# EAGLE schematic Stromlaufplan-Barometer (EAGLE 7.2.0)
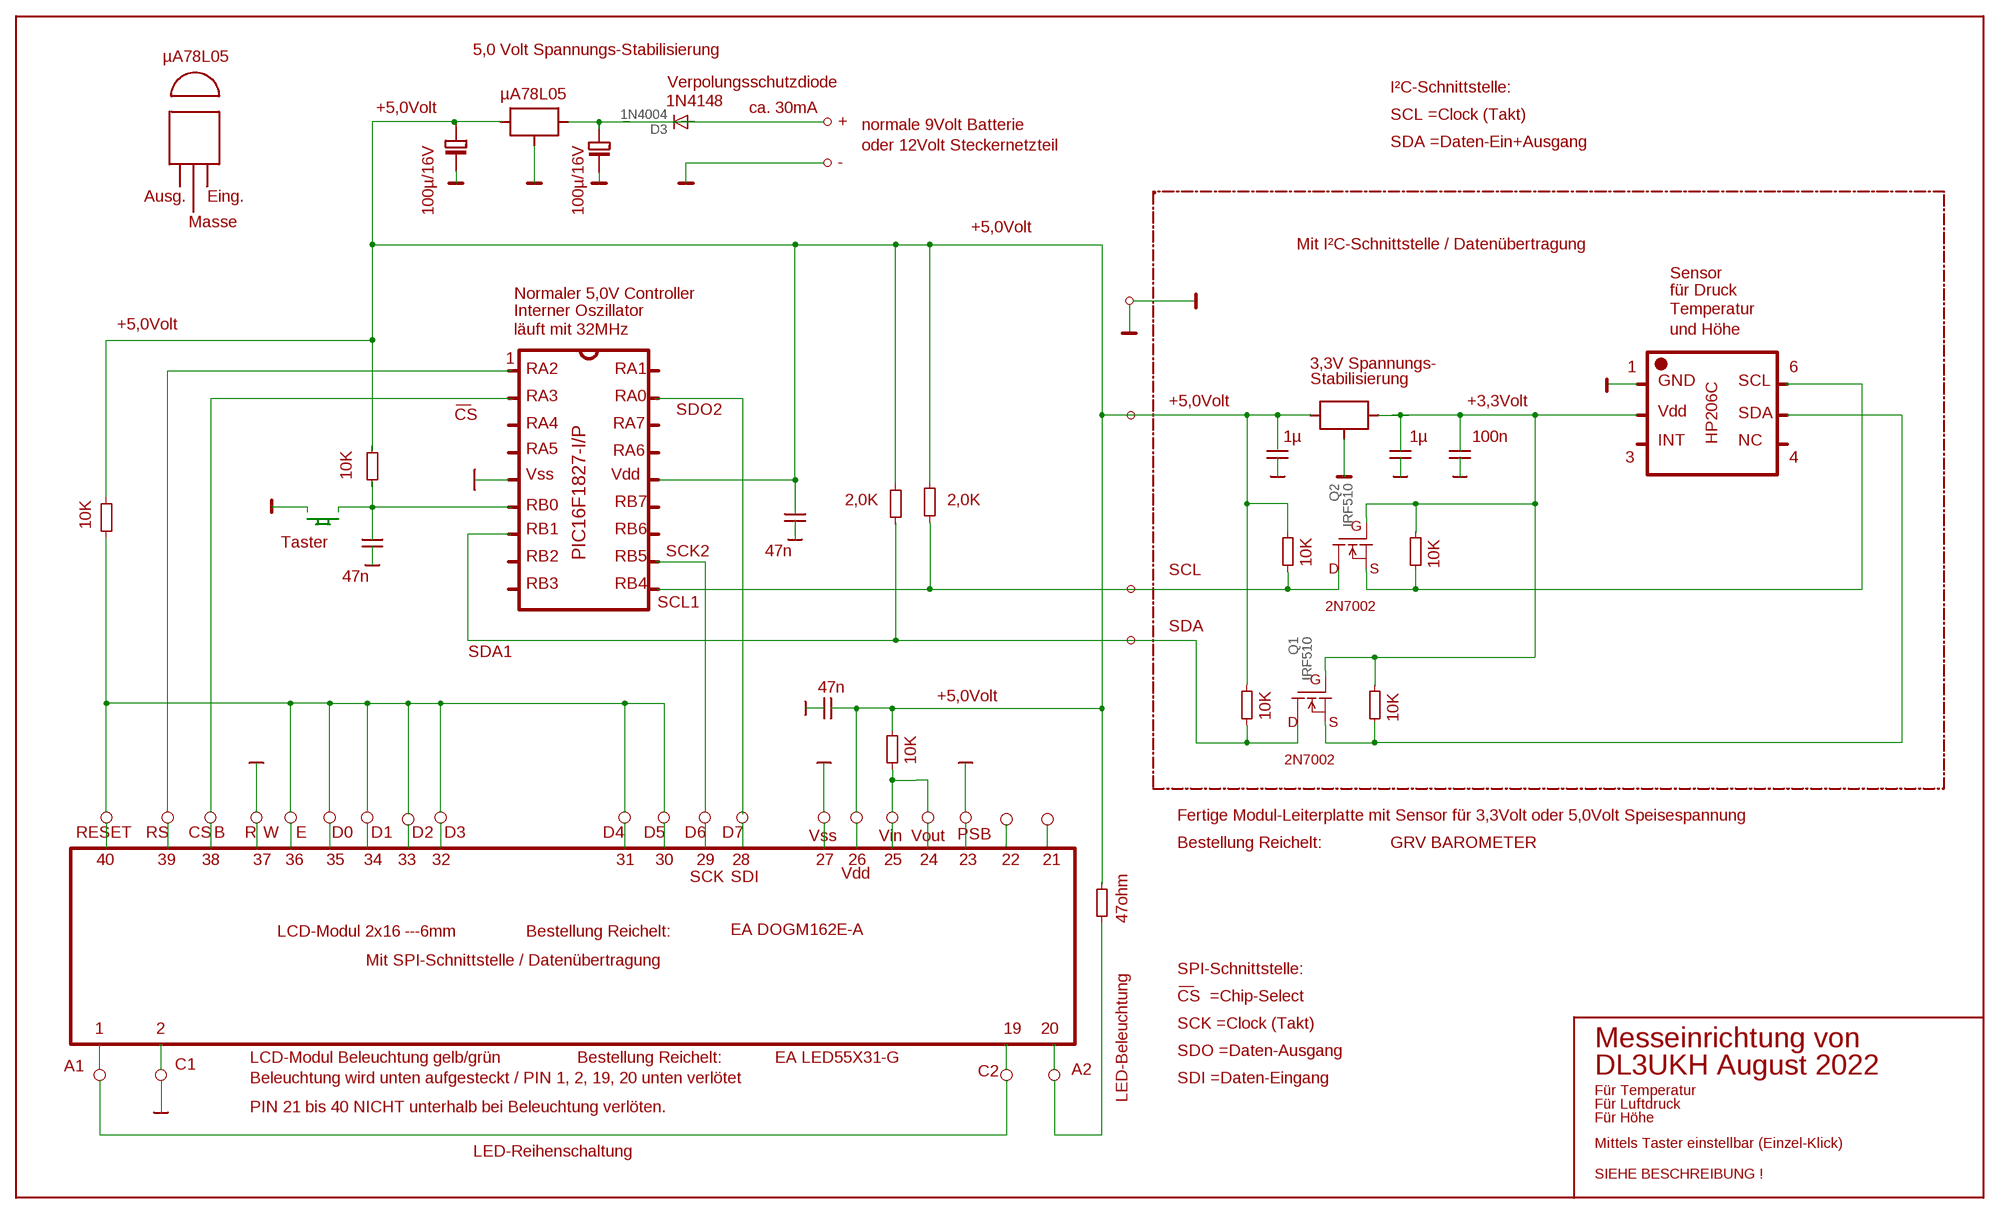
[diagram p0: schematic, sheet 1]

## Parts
D3  1N4004  [DO41-10]
Q1  IRF510  [TO220]
Q2  IRF510  [TO220]

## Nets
N$21: Q2.2(D)
N$22: Q1.3(S)
N$23: Q1.2(D)
N$30: Q1.1(G)
N$35: D3.C
N$47: D3.A
N$55: Q2.1(G)
N$71: Q2.3(S)

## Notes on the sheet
- 5,0 Volt Spannungs-Stabilisierung
- µA78L05
- Verpolungsschutzdiode
- I²C-Schnittstelle:
- µA78L05
- 1N4148
- +5,0Volt | ca. 30mA
- SCL =Clock (Takt)
- + | normale 9Volt Batterie
- oder 12Volt Steckernetzteil | SDA =Daten-Ein+Ausgang
- -
- Ausg. | Eing.
- 100µ/16V | 100µ/16V
- Masse
- +5,0Volt
- Mit I²C-Schnittstelle / Datenübertragung
- Sensor
- Normaler 5,0V Controller | für Druck
- Interner Oszillator | Temperatur
- +5,0Volt
- läuft mit 32MHz | und Höhe
- 1
- 3,3V Spannungs- | 1 | 6
- RA2 | RA1
- Stabilisierung | GND | SCL
- RA3 | RA0
- +5,0Volt | +3,3Volt
- SDO2 | Vdd | SDA
- CS
- RA4 | RA7 | 1µ | 1µ | 100n
- INT | HP206C | NC
- RA5 | RA6
- 3 | 4
- 10K | Vss | Vdd
- RB7 | 2,0K | 2,0K
- RB0
- G
- 10K
- Taster | RB1 | RB6
- 47n
- PIC16F1827-I/P | SCK2
- RB2 | RB5 | D | S
- 47n | 10K | 10K
- SCL
- RB3 | RB4
- 2N7002
- SCL1
- SDA
- SDA1
- G
- 47n
- +5,0Volt
- 10K | D | S
- 10K
- 2N7002
- 10K
- Fertige Modul-Leiterplatte mit Sensor für 3,3Volt oder 5,0Volt Speisespannung
- RESET | RS | CS | B | R | W | E | D0 | D1 | D2 | D3 | D4 | D5 | D6 | D7 | Vss | Vin | Vout | PSB
- Bestellung Reichelt: | GRV BAROMETER
- 40 | 39 | 38 | 37 | 36 | 35 | 34 | 33 | 32 | 31 | 30 | 29 | 28 | 27 | 26 | 25 | 24 | 23 | 22 | 21
- SCK | SDI | Vdd
- 47ohm
- LCD-Modul 2x16 ---6mm | Bestellung Reichelt: | EA DOGM162E-A
- Mit SPI-Schnittstelle / Datenübertragung
- SPI-Schnittstelle:
- CS  =Chip-Select
- SCK =Clock (Takt)
- 1 | 2 | 19 | 20
- Messeinrichtung von
- SDO =Daten-Ausgang
- LCD-Modul Beleuchtung gelb/grün | Bestellung Reichelt: | EA LED55X31-G
- A1 | C1
- C2 | A2 | DL3UKH August 2022
- Beleuchtung wird unten aufgesteckt / PIN 1, 2, 19, 20 unten verlötet | SDI =Daten-Eingang
- Für Temperatur
- LED-Beleuchtung
- PIN 21 bis 40 NICHT unterhalb bei Beleuchtung verlöten. | Für Luftdruck
- Für Höhe
- Mittels Taster einstellbar (Einzel-Klick)
- LED-Reihenschaltung
- SIEHE BESCHREIBUNG !

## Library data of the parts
D3 = diode:1N4004: DIODE
Q1 Q2 = transistor-fet:IRF510: N-Channel Enhancement MOSFET (HEXFET); 100V; 5,6A; 0,54Ohm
